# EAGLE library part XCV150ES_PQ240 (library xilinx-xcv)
xcv150es_pq240 edit this description Auto generated by make-symbol-device-package-bsdl.ulp Rev. 26 Source: xcv150es_pq240.bsd
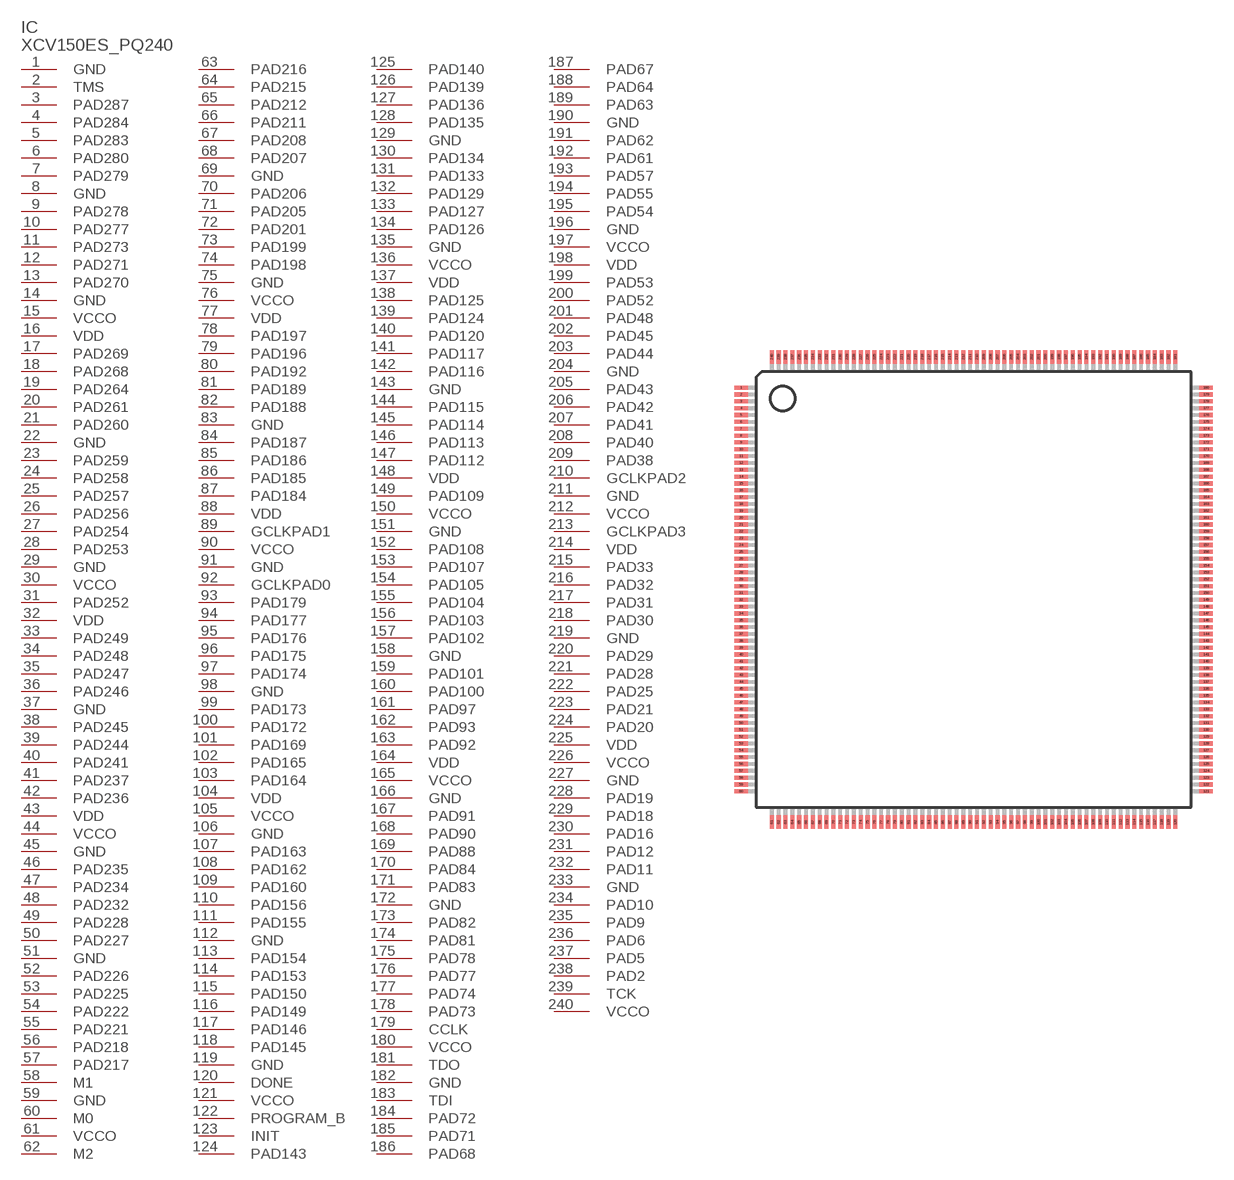
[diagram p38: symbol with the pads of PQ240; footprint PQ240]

Designator prefix IC

## XCV150ES_PQ240 (OC_FARNELL: unknown; OC_NEWARK: unknown)  [PQ240]
1  GND  pwr
2  TMS  in
3  PAD287
4  PAD284
5  PAD283
6  PAD280
7  PAD279
8  GND  pwr
9  PAD278
10  PAD277
11  PAD273
12  PAD271
13  PAD270
14  GND  pwr
15  VCCO  pwr
16  VDD  pwr
17  PAD269
18  PAD268
19  PAD264
20  PAD261
21  PAD260
22  GND  pwr
23  PAD259
24  PAD258
25  PAD257
26  PAD256
27  PAD254
28  PAD253
29  GND  pwr
30  VCCO  pwr
31  PAD252
32  VDD  pwr
33  PAD249
34  PAD248
35  PAD247
36  PAD246
37  GND  pwr
38  PAD245
39  PAD244
40  PAD241
41  PAD237
42  PAD236
43  VDD  pwr
44  VCCO  pwr
45  GND  pwr
46  PAD235
47  PAD234
48  PAD232
49  PAD228
50  PAD227
51  GND  pwr
52  PAD226
53  PAD225
54  PAD222
55  PAD221
56  PAD218
57  PAD217
58  M1  in
59  GND  pwr
60  M0  in
61  VCCO  pwr
62  M2  in
63  PAD216
64  PAD215
65  PAD212
66  PAD211
67  PAD208
68  PAD207
69  GND  pwr
70  PAD206
71  PAD205
72  PAD201
73  PAD199
74  PAD198
75  GND  pwr
76  VCCO  pwr
77  VDD  pwr
78  PAD197
79  PAD196
80  PAD192
81  PAD189
82  PAD188
83  GND  pwr
84  PAD187
85  PAD186
86  PAD185
87  PAD184
88  VDD  pwr
89  GCLKPAD1  in
90  VCCO  pwr
91  GND  pwr
92  GCLKPAD0  in
93  PAD179
94  PAD177
95  PAD176
96  PAD175
97  PAD174
98  GND  pwr
99  PAD173
100  PAD172
101  PAD169
102  PAD165
103  PAD164
104  VDD  pwr
105  VCCO  pwr
106  GND  pwr
107  PAD163
108  PAD162
109  PAD160
110  PAD156
111  PAD155
112  GND  pwr
113  PAD154
114  PAD153
115  PAD150
116  PAD149
117  PAD146
118  PAD145
119  GND  pwr
120  DONE
121  VCCO  pwr
122  PROGRAM_B  in
123  INIT
124  PAD143
125  PAD140
126  PAD139
127  PAD136
128  PAD135
129  GND  pwr
130  PAD134
131  PAD133
132  PAD129
133  PAD127
134  PAD126
135  GND  pwr
136  VCCO  pwr
137  VDD  pwr
138  PAD125
139  PAD124
140  PAD120
141  PAD117
142  PAD116
143  GND  pwr
144  PAD115
145  PAD114
146  PAD113
147  PAD112
148  VDD  pwr
149  PAD109
150  VCCO  pwr
151  GND  pwr
152  PAD108
153  PAD107
154  PAD105
155  PAD104
156  PAD103
157  PAD102
158  GND  pwr
159  PAD101
160  PAD100
161  PAD97
162  PAD93
163  PAD92
164  VDD  pwr
165  VCCO  pwr
166  GND  pwr
167  PAD91
168  PAD90
169  PAD88
170  PAD84
171  PAD83
172  GND  pwr
173  PAD82
174  PAD81
175  PAD78
176  PAD77
177  PAD74
178  PAD73
179  CCLK
180  VCCO  pwr
181  TDO  out
182  GND  pwr
183  TDI  in
184  PAD72
185  PAD71
186  PAD68
187  PAD67
188  PAD64
189  PAD63
190  GND  pwr
191  PAD62
192  PAD61
193  PAD57
194  PAD55
195  PAD54
196  GND  pwr
197  VCCO  pwr
198  VDD  pwr
199  PAD53
200  PAD52
201  PAD48
202  PAD45
203  PAD44
204  GND  pwr
205  PAD43
206  PAD42
207  PAD41
208  PAD40
209  PAD38
210  GCLKPAD2  in
211  GND  pwr
212  VCCO  pwr
213  GCLKPAD3  in
214  VDD  pwr
215  PAD33
216  PAD32
217  PAD31
218  PAD30
219  GND  pwr
220  PAD29
221  PAD28
222  PAD25
223  PAD21
224  PAD20
225  VDD  pwr
226  VCCO  pwr
227  GND  pwr
228  PAD19
229  PAD18
230  PAD16
231  PAD12
232  PAD11
233  GND  pwr
234  PAD10
235  PAD9
236  PAD6
237  PAD5
238  PAD2
239  TCK  in
240  VCCO  pwr

## Footprint PQ240 (pad centres in mm)
PQ240 Auto generated by make-symbol-device-package-bsdl.ulp Rev. 26
smd 1 x 0.3: 1 -17,14.75; 2 -17,14.25; 3 -17,13.75; 4 -17,13.25; 5 -17,12.75; 6 -17,12.25; 7 -17,11.75; 8 -17,11.25; 9 -17,10.75; 10 -17,10.25; 11 -17,9.75; 12 -17,9.25; 13 -17,8.75; 14 -17,8.25; 15 -17,7.75; 16 -17,7.25; 17 -17,6.75; 18 -17,6.25; 19 -17,5.75; 20 -17,5.25; 21 -17,4.75; 22 -17,4.25; 23 -17,3.75; 24 -17,3.25; 25 -17,2.75; 26 -17,2.25; 27 -17,1.75; 28 -17,1.25; 29 -17,0.75; 30 -17,0.25; 31 -17,-0.25; 32 -17,-0.75; 33 -17,-1.25; 34 -17,-1.75; 35 -17,-2.25; 36 -17,-2.75; 37 -17,-3.25; 38 -17,-3.75; 39 -17,-4.25; 40 -17,-4.75; 41 -17,-5.25; 42 -17,-5.75; 43 -17,-6.25; 44 -17,-6.75; 45 -17,-7.25; 46 -17,-7.75; 47 -17,-8.25; 48 -17,-8.75; 49 -17,-9.25; 50 -17,-9.75; 51 -17,-10.25; 52 -17,-10.75; 53 -17,-11.25; 54 -17,-11.75; 55 -17,-12.25; 56 -17,-12.75; 57 -17,-13.25; 58 -17,-13.75; 59 -17,-14.25; 60 -17,-14.75; 121 17,-14.75; 122 17,-14.25; 123 17,-13.75; 124 17,-13.25; 125 17,-12.75; 126 17,-12.25; 127 17,-11.75; 128 17,-11.25; 129 17,-10.75; 130 17,-10.25; 131 17,-9.75; 132 17,-9.25; 133 17,-8.75; 134 17,-8.25; 135 17,-7.75; 136 17,-7.25; 137 17,-6.75; 138 17,-6.25; 139 17,-5.75; 140 17,-5.25; 141 17,-4.75; 142 17,-4.25; 143 17,-3.75; 144 17,-3.25; 145 17,-2.75; 146 17,-2.25; 147 17,-1.75; 148 17,-1.25; 149 17,-0.75; 150 17,-0.25; 151 17,0.25; 152 17,0.75; 153 17,1.25; 154 17,1.75; 155 17,2.25; 156 17,2.75; 157 17,3.25; 158 17,3.75; 159 17,4.25; 160 17,4.75; 161 17,5.25; 162 17,5.75; 163 17,6.25; 164 17,6.75; 165 17,7.25; 166 17,7.75; 167 17,8.25; 168 17,8.75; 169 17,9.25; 170 17,9.75; 171 17,10.25; 172 17,10.75; 173 17,11.25; 174 17,11.75; 175 17,12.25; 176 17,12.75; 177 17,13.25; 178 17,13.75; 179 17,14.25; 180 17,14.75
smd 0.3 x 1: 61 -14.75,-17; 62 -14.25,-17; 63 -13.75,-17; 64 -13.25,-17; 65 -12.75,-17; 66 -12.25,-17; 67 -11.75,-17; 68 -11.25,-17; 69 -10.75,-17; 70 -10.25,-17; 71 -9.75,-17; 72 -9.25,-17; 73 -8.75,-17; 74 -8.25,-17; 75 -7.75,-17; 76 -7.25,-17; 77 -6.75,-17; 78 -6.25,-17; 79 -5.75,-17; 80 -5.25,-17; 81 -4.75,-17; 82 -4.25,-17; 83 -3.75,-17; 84 -3.25,-17; 85 -2.75,-17; 86 -2.25,-17; 87 -1.75,-17; 88 -1.25,-17; 89 -0.75,-17; 90 -0.25,-17; 91 0.25,-17; 92 0.75,-17; 93 1.25,-17; 94 1.75,-17; 95 2.25,-17; 96 2.75,-17; 97 3.25,-17; 98 3.75,-17; 99 4.25,-17; 100 4.75,-17; 101 5.25,-17; 102 5.75,-17; 103 6.25,-17; 104 6.75,-17; 105 7.25,-17; 106 7.75,-17; 107 8.25,-17; 108 8.75,-17; 109 9.25,-17; 110 9.75,-17; 111 10.25,-17; 112 10.75,-17; 113 11.25,-17; 114 11.75,-17; 115 12.25,-17; 116 12.75,-17; 117 13.25,-17; 118 13.75,-17; 119 14.25,-17; 120 14.75,-17; 181 14.75,17; 182 14.25,17; 183 13.75,17; 184 13.25,17; 185 12.75,17; 186 12.25,17; 187 11.75,17; 188 11.25,17; 189 10.75,17; 190 10.25,17; 191 9.75,17; 192 9.25,17; 193 8.75,17; 194 8.25,17; 195 7.75,17; 196 7.25,17; 197 6.75,17; 198 6.25,17; 199 5.75,17; 200 5.25,17; 201 4.75,17; 202 4.25,17; 203 3.75,17; 204 3.25,17; 205 2.75,17; 206 2.25,17; 207 1.75,17; 208 1.25,17; 209 0.75,17; 210 0.25,17; 211 -0.25,17; 212 -0.75,17; 213 -1.25,17; 214 -1.75,17; 215 -2.25,17; 216 -2.75,17; 217 -3.25,17; 218 -3.75,17; 219 -4.25,17; 220 -4.75,17; 221 -5.25,17; 222 -5.75,17; 223 -6.25,17; 224 -6.75,17; 225 -7.25,17; 226 -7.75,17; 227 -8.25,17; 228 -8.75,17; 229 -9.25,17; 230 -9.75,17; 231 -10.25,17; 232 -10.75,17; 233 -11.25,17; 234 -11.75,17; 235 -12.25,17; 236 -12.75,17; 237 -13.25,17; 238 -13.75,17; 239 -14.25,17; 240 -14.75,17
